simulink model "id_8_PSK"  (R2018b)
settings: Solver=VariableStepAuto  StartTime=0.0  StopTime=inf  RelTol=1e-3
libraries: commdigbbndpm3 x2, commfilt2 x2, commchan3 x1, commrandsrc3 x1, commsink2 x1, commutil2 x1

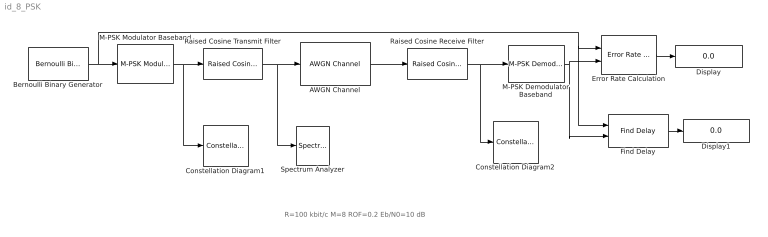
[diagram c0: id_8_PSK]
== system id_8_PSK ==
  note: R=100 kbit/c M=8 ROF=0.2 Eb/N0=10 dB
  AWGN Channel : commchan3/AWGN Channel  InputProcessing=Columns as channels (frame based)  seed=67  noiseMode="Signal to noise ratio  (Eb/No)"  EbNodB=10  EsNodB=10  SNRdB=10  bitsPerSym=3  Ps=1/8  Tsym=1/300e3  variance=1
  Bernoulli Binary Generator : commrandsrc3/Bernoulli Binary Generator  ProbabilityOfZero=0.5  SeedSource=Auto  Seed=0  SampleTime=1/900e3  SamplesPerFrame=300  OutputDataType=double  SimulateUsing=Interpreted execution
  Constellation Diagram1 : ConstellationDiagram
  Constellation Diagram2 : ConstellationDiagram
  Display : Display
  Display1 : Display
  Error Rate Calculation : commsink2/Error Rate Calculation  N=30  st_delay=0  cp_mode=Entire frame  subframe=[]  PMode=Port  WsName=ErrorVec  RsMode2=off  stop=off  numErr=100  maxBits=1e6
  Find Delay : commutil2/Find Delay  corrLength=200  chgSigOP=off  stopUpdate=off  numConstDelay=3
  M-PSK Demodulator Baseband : commdigbbndpm3/M-PSK Demodulator Baseband  M=8  OutType=Bit  DecType=Hard decision  VarSource=Dialog  Variance=1  Dec=Gray  Mapping=[0:7]  Ph=pi/8  outDtype1=Inherit via internal rule  outDtype2=Inherit via internal rule  derotateFactorWordLen=16  derotateFactorDataTypeStr=Inherit: Same word length as input  derotateFactorLastDataTypeStr=Inherit: Same word length as input
  M-PSK Modulator Baseband : commdigbbndpm3/M-PSK Modulator Baseband  M=8  InType=Bit  Enc=Gray  Mapping=[0:7]  Ph=pi/8  outDtype=double  outWordLen=16  outUDDataType=sfix(16)  outFracLenMode=Best precision  outFracLen=15  outDataTypeStr=double  outLastDataTypeStr=double
  Raised Cosine Receive Filter : commfilt2/Raised Cosine Receive Filter  filtType=Square root  R=0.2  filtSpan=10  N=8  downFactor=8  downOffset=0  filterGain=1  InputProcessing=Columns as channels (frame based)  RateOptions=Enforce single-rate processing  framing=Mute  checkCoeff=off  variableName=rcRxFilt  currentFiltSpan=10  D=5  inputOffset=0  sampMode=Mute  saveAsFlag=0  rateMode=Downsampling  checkGain=Normalized  launchFVT=on  roundingMode=Floor  overflowMode=off  coeffDataTypeStr=Inherit: Same word length as input  coeffMin=[]  coeffMax=[]  coeffLastDataTypeStr=Inherit: Same word length as input  accumDataTypeStr=Inherit: Same as product output  accumLastDataTypeStr=Inherit: Same as product output  outputDataTypeStr=Inherit: Same as accumulator  outputMin=[]  outputMax=[]  outputLastDataTypeStr=Inherit: Same as accumulator
  Raised Cosine Transmit Filter : commfilt2/Raised Cosine Transmit Filter  filtType=Square root  R=0.2  filtSpan=10  N=8  filterGain=1  InputProcessing=Columns as channels (frame based)  RateOptions=Enforce single-rate processing  framing=Mute  checkCoeff=off  variableName=rcTxFilt  checkGain=Normalized  sampMode=Mute  saveAsFlag=0  currentFiltSpan=10  D=(10)/2  launchFVT=on  roundingMode=Floor  overflowMode=off  coeffDataTypeStr=Inherit: Same word length as input  coeffMin=[]  coeffMax=[]  coeffLastDataTypeStr=Inherit: Same word length as input  outputDataTypeStr=Inherit: Same as accumulator  outputMin=[]  outputMax=[]  outputLastDataTypeStr=Inherit: Same as accumulator
  Spectrum Analyzer : SpectrumAnalyzer
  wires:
  Bernoulli Binary Generator/1 -> Find Delay/1, Error Rate Calculation/1, M-PSK Modulator Baseband/1
  M-PSK Modulator Baseband/1 -> Constellation Diagram1/1, Raised Cosine Transmit Filter/1
  Raised Cosine Transmit Filter/1 -> AWGN Channel/1, Spectrum Analyzer/1
  AWGN Channel/1 -> Raised Cosine Receive Filter/1
  Raised Cosine Receive Filter/1 -> Constellation Diagram2/1, M-PSK Demodulator Baseband/1
  M-PSK Demodulator Baseband/1 -> Find Delay/2, Error Rate Calculation/2
  Find Delay/1 -> Display1/1
  Error Rate Calculation/1 -> Display/1
